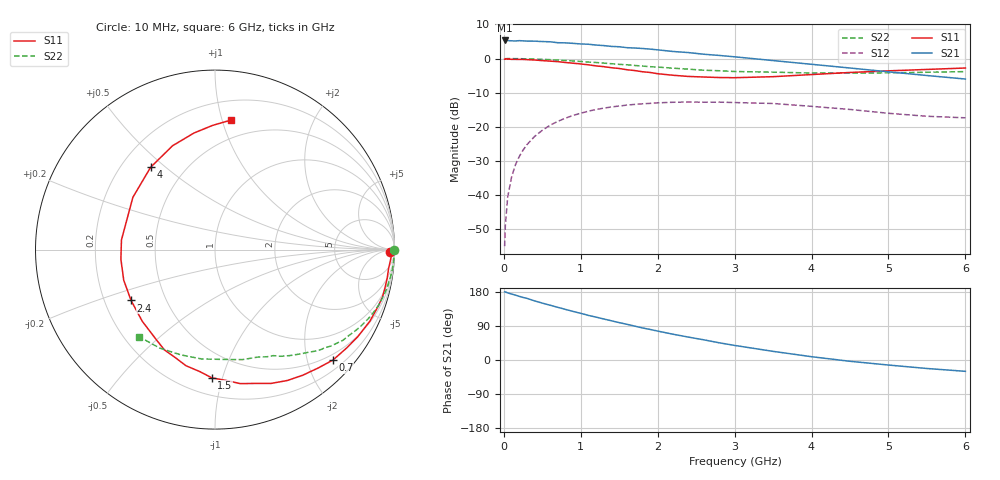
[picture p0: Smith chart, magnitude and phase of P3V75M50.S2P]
! SIEMENS Small Signal Semiconductors
! BFP181
! Si NPN RF Bipolar Junction Transistor in SOT143
! VCE = 0.75 V  IC = 0.5 mA
! Common Emitter S-Parameters:  March  1996
# GHz  S  MA  R  50
!  f  S11  S21  S12  S22
! GHz  MAG  ANG  MAG  ANG  MAG  ANG  MAG  ANG
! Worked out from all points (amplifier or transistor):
!   36 points, 10 MHz to 6 GHz, reference 50 ohm
!   highest |S21| = 5.3 dB at 10 MHz (marker M1)
!   |S21| within 3 dB of that: start of sweep to 2.106 GHz
!   unconditionally stable (mu >= 1): 3.546 GHz to end of sweep
!   at 250 MHz: K = 0.09, MSG = 16.0 dB, |S12| = -26.8 dB
!   at 1.4 GHz: K = 0.48, MSG = 8.9 dB, |S12| = -14.2 dB
!   at 6 GHz: K = 1.61, MAG = 1.1 dB, |S12| = -17.3 dB
!   S11 on the Smith chart (normalised r, x): 10 MHz: 62, -36; 700 MHz: 0.38, -2.48; 1.5 GHz: 0.32, -0.92; 2.4 GHz: 0.31, -0.25; 4 GHz: 0.32, +0.45; 6 GHz: 0.35, +1.07
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0.01  0.9764 -0.8  1.837 179.8  0.0018 89.2  0.9997 -0.2
0.02  0.9833 -1.2  1.82 179.6  0.0037 89.3  0.992 -0.6
0.05  0.9811 -2.9  1.829 177.2  0.0094 90.0  0.9977 -1.6
0.1  0.9728 -6.3  1.815 174.2  0.0183 84.9  0.9978 -3.2
0.15  0.9725 -9.4  1.804 171.2  0.0278 82.6  0.9957 -4.8
0.25  0.9697 -15.7  1.813 165.0  0.0457 78.8  0.9913 -8.0
0.4  0.9507 -24.8  1.795 156.0  0.0725 72.4  0.9816 -12.7
0.6  0.9156 -36.8  1.757 144.6  0.1056 63.3  0.9622 -18.9
0.7  0.9003 -43.1  1.703 139.1  0.1203 59.3  0.9493 -21.8
0.9  0.8537 -55.1  1.666 128.2  0.147 50.9  0.92 -27.3
1.1  0.8083 -67.3  1.617 117.7  0.1698 43.3  0.8874 -32.5
1.5  0.7148 -91.4  1.486 98.6  0.2017 29.6  0.8213 -41.7
1.9  0.6257 -116.8  1.373 80.7  0.2207 17.8  0.7598 -49.5
2.2  0.569 -135.4  1.267 68.0  0.2291 10.2  0.7228 -54.8
2.4  0.5468 -148.8  1.221 60.4  0.2309 5.1  0.6986 -58.3
2.8  0.527 -174.2  1.109 45.4  0.2301 -3.1  0.6625 -64.4
3  0.524 174.1  1.059 38.5  0.227 -7.6  0.6458 -67.8
3.5  0.5424 147.5  0.933 22.8  0.2199 -15.7  0.6318 -76.0
4  0.5824 128.0  0.823 8.7  0.1997 -22.6  0.6133 -86.0
4.5  0.6251 112.2  0.726 -3.4  0.1799 -28.0  0.6138 -96.9
5.5  0.6921 91.1  0.564 -22.4  0.143 -27.9  0.6294 -119.4
6  0.7264 83.1  0.501 -29.9  0.1357 -24.2  0.6434 -131.0
